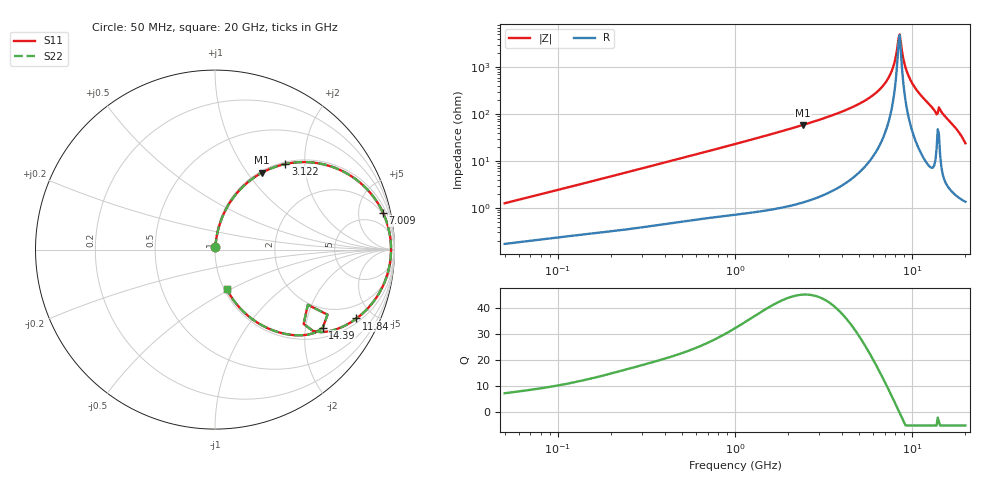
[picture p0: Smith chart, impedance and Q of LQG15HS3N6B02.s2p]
!Murata Part Number: LQG15HS3N6B02
!These Parameters are Measured in Series Mode Connection
!  o--[Z]--o
!Port1  Port2
!  o-------o
!Freq. Start=50[MHz] Stop=20[GHz], 401[Steps]
# Hz S RI R 50
!Freq.(Hz) S11(Real) S11(Imag) S21(Real) S21(Imag) S12(Real) S12(Imag) S22(Real) S22(Imag)
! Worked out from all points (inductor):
!   401 points, 50 MHz to 20 GHz, reference 50 ohm
!   read as one part in series: L = 3.91 nH near 51.52 MHz
!   highest Q = 44.9 at 2.42 GHz (marker M1), where L = 3.86 nH
!   self-resonance near 8.389 GHz
!   S11 on the Smith chart (normalised r, x): 50 MHz: 1.00, +0.02; 3.122 GHz: 1.04, +1.60; 7.009 GHz: 1.77, +8.92; 11.84 GHz: 1.20, -4.00; 14.39 GHz: 1.29, -2.49; 20 GHz: 1.03, -0.48
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5e7  0.00186 0.0124  0.9981 -0.0124  0.9981 -0.0124  0.00186 0.0124
1.364002e8  0.00372 0.0323  0.9963 -0.0323  0.9963 -0.0323  0.00372 0.0323
3.721004e8  0.0116 0.0849  0.9884 -0.0849  0.9884 -0.0849  0.0116 0.0849
1e9  0.0562 0.2152  0.9438 -0.2152  0.9438 -0.2152  0.0562 0.2152
2.419936e9  0.261 0.4282  0.739 -0.4282  0.739 -0.4282  0.261 0.4282
2.728004e9  0.3172 0.4543  0.6828 -0.4543  0.6828 -0.4543  0.3172 0.4543
3.121702e9  0.3914 0.4767  0.6086 -0.4767  0.6086 -0.4767  0.3914 0.4767
5.194772e9  0.7505 0.415  0.2495 -0.415  0.2495 -0.415  0.7505 0.415
7.009217e9  0.9365 0.2046  0.0635 -0.2046  0.0635 -0.2046  0.9365 0.2046
7.442007e9  0.9592 0.1453  0.0408 -0.1453  0.0408 -0.1453  0.9592 0.1453
7.901521e9  0.9744 0.0812  0.0256 -0.0812  0.0256 -0.0812  0.9744 0.0812
8.264682e9  0.98 0.0304  0.02 -0.0304  0.02 -0.0304  0.98 0.0304
8.516016e9  0.9808 -0.00456  0.0192 0.00456  0.0192 0.00456  0.9808 -0.00456
8.644534e9  0.9803 -0.0223  0.0197 0.0223  0.0197 0.0223  0.9803 -0.0223
9.178299e9  0.9712 -0.0945  0.0288 0.0945  0.0288 0.0945  0.9712 -0.0945
9.600142e9  0.9567 -0.1492  0.0433 0.1492  0.0433 0.1492  0.9567 -0.1492
1.050288e10  0.9059 -0.2567  0.0941 0.2567  0.0941 0.2567  0.9059 -0.2567
1.183995e10  0.7882 -0.3837  0.2118 0.3837  0.2118 0.3837  0.7882 -0.3837
1.354865e10  0.545 -0.4527  0.455 0.4527  0.455 0.4527  0.545 -0.4527
1.438523e10  0.5998 -0.436  0.4002 0.436  0.4002 0.436  0.5998 -0.436
1.621653e10  0.3445 -0.4575  0.6555 0.4575  0.6555 0.4575  0.3445 -0.4575
2e10  0.0651 -0.2199  0.9349 0.2199  0.9349 0.2199  0.0651 -0.2199
